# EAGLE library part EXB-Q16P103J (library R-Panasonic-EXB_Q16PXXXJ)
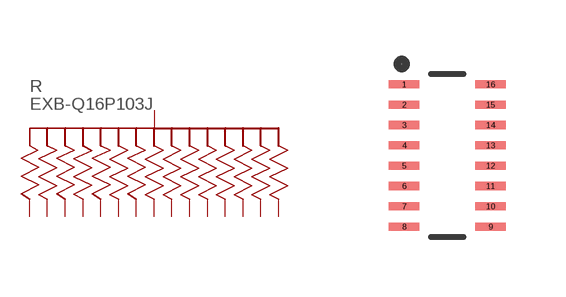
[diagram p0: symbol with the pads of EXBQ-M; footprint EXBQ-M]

Designator prefix R

## EXB-Q16P103JEXBQ-M (MANUFACTURER_PART_NUMBER: EXBQ16P103J; VENDOR: Panasonic)  [EXBQ-M]
1  1  pas
2  3  pas
3  5  pas
4  7  pas
5  9  pas
6  11  pas
7  13  pas
8  15  pas
9  14  pas
10  12  pas
11  10  pas
12  8  pas
13  6  pas
14  4  pas
15  2  pas
16  COM  pas

## Footprint EXBQ-M (pad centres in mm)
smd 0.762 x 0.203: 1 -1.079,1.778; 2 -1.079,1.27; 3 -1.079,0.762; 4 -1.079,0.254; 5 -1.079,-0.254; 6 -1.079,-0.762; 7 -1.079,-1.27; 8 -1.079,-1.778; 9 1.079,-1.778; 10 1.079,-1.27; 11 1.079,-0.762; 12 1.079,-0.254; 13 1.079,0.254; 14 1.079,0.762; 15 1.079,1.27; 16 1.079,1.778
